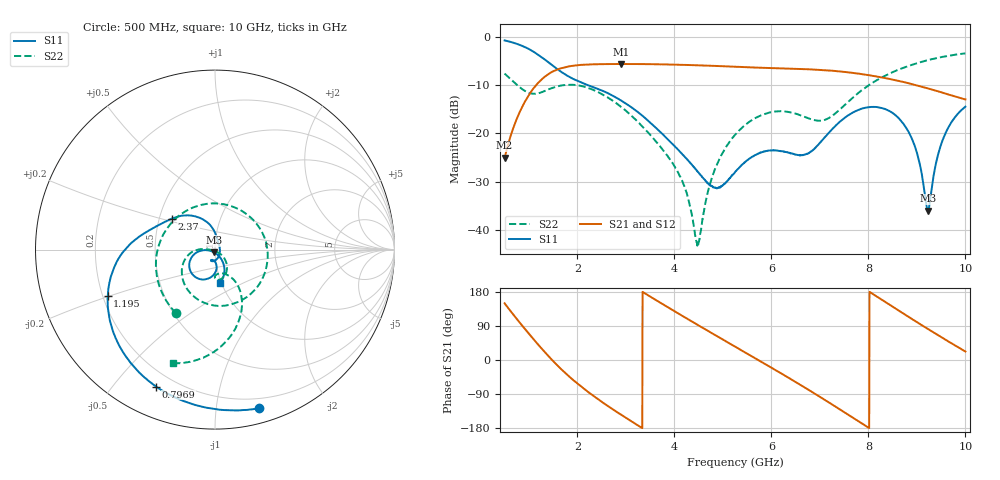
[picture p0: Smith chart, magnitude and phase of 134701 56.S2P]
!  2-Port S-parameters saved by WinCal
! VAR MeasName=S-Parameters (CALIBRATED_DATA) read from VNA (N5242A)
! VAR MeasDate=2013-7-3 16:40:19
! VAR NAME=134701 56
! VAR FILENAME=134701 56.S2P
! VAR DATE=2013-7-3 16:40:19
! VAR PHYS_PORTS=1,2
# Hz S MA R 50
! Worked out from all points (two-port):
!   1601 points, 500 MHz to 10 GHz, reference 50 ohm
!   highest |S21| = -5.62 dB at 2.905 GHz (marker M1); lowest = -25.0 dB at 500 MHz (marker M2)
!   |S21| within 3 dB of the highest: 1.286 GHz to 8.386 GHz (7.1 GHz wide, 147 % of centre)
!   lowest |S11| = -36.0 dB at 9.228 GHz (marker M3), VSWR 1.03, Z = 49.3 - j1.4 ohm
!   |S11| at or under -10 dB: 2.213 GHz to end of sweep
!   |S22| runs from -43.4 to -3.4 dB; largest |S21 - S12| = 0.0023
!   S11 on the Smith chart (normalised r, x): 500 MHz: 0.12, -1.31; 796.9 MHz: 0.13, -0.65; 1.195 GHz: 0.22, -0.20; 2.37 GHz: 0.58, +0.22; 10 GHz: 0.98, -0.38
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5e8  0.9178 -74.6  0.05597 149.7  0.05599 149.3  0.4163 -121.7
7.96875e8  0.831 -113.2  0.16 101.0  0.1598 100.9  0.3047 167.9
9.9875e8  0.7483 -136.7  0.2489 69.8  0.2486 69.7  0.263 114.1
1.194688e9  0.6514 -156.6  0.3348 40.3  0.3347 40.2  0.2604 60.6
1.396562e9  0.5495 -173.3  0.4096 11.5  0.4094 11.4  0.2852 12.0
1.604375e9  0.4568 174.0  0.4627 -16.4  0.462 -16.5  0.3078 -28.1
2.085312e9  0.3362 155.1  0.5126 -70.9  0.5119 -71.0  0.3093 -93.6
2.370312e9  0.2955 144.3  0.5198 -98.4  0.5187 -98.4  0.2761 -121.2
2.904688e9  0.2185 121.5  0.5235 -144.7  0.5221 -144.8  0.1878 -158.3
3.670625e9  0.1078 93.5  0.5203 154.2  0.5195 154.3  0.07687 178.3
4.187188e9  0.05915 77.4  0.5122 114.7  0.5116 114.8  0.0296 -178.2
4.478125e9  0.04014 60.1  0.5066 92.8  0.5075 92.8  0.007014 -112.1
4.79875e9  0.02755 17.0  0.5007 68.9  0.5007 68.9  0.03777 -39.6
5.25e9  0.03951 -54.9  0.4902 35.3  0.4907 35.3  0.09649 -49.3
5.992188e9  0.06648 -104.1  0.4747 -19.6  0.4746 -19.7  0.1658 -76.8
6.835312e9  0.0656 -91.9  0.4595 -84.2  0.4594 -84.2  0.1392 -86.6
7.678438e9  0.1643 -102.2  0.4229 -151.9  0.4237 -152.1  0.2338 -57.5
8.420625e9  0.1717 -146.6  0.368 147.2  0.3673 147.0  0.4124 -70.9
8.9075e9  0.08551 -174.7  0.3233 107.5  0.3227 107.2  0.515 -83.1
9.228125e9  0.01581 -115.9  0.2921 81.7  0.2918 81.6  0.5737 -91.2
9.530938e9  0.08518 -58.3  0.2638 58.0  0.2631 57.7  0.6205 -98.9
1e10  0.1889 -81.6  0.2248 22.4  0.2244 22.3  0.6745 -110.2
